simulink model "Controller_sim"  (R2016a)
settings: Solver=FixedStepAuto  StartTime=0.0  StopTime=Endtime  FixedStep=0.05  RelTol=1e-3
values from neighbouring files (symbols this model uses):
  alpha_A = (2^n - 1)/(V_A_max - V_A_min)    (= 204.6)    [Controller.m]    (also in ADConverter.m)
  alpha_i = 5/37.5    (= 0.133333333333)    [Controller.m]    (also in MotorDriver.m)
  alpha_T = 1.5/1000    (= 0.0015)    [Controller.m]    (also in Tachogenerator.m)
  d_i_d = (2^n-1)/60    (= 17.05)    [Controller.m]
  d_N_d = (2^n-1)/60    (= 17.05)    [Controller.m]
  m = 8    [Controller.m]    (also in PulseGenerator.m)
  u_max = 100    [Controller.m]    (also in SystemModel_noise1.m; SystemModel_noise2.m)
  u_min = 0    [Controller.m]    (also in SystemModel_noise1.m; SystemModel_noise2.m)
  V_A_min = 0    [Controller.m]    (also in ADConverter.m)
libraries: simulink x2

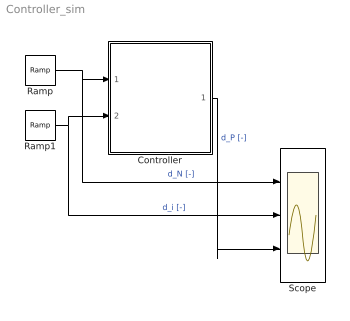
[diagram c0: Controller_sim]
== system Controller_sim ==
  Controller : Subsystem
  Ramp : simulink/Sources/Ramp  slope=d_N_d  start=0  X0=0
  Ramp1 : simulink/Sources/Ramp  slope=d_i_d  start=0  X0=0
  Scope : Scope  NumInputPorts=3
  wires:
  Ramp/1 -> Controller/1(d_N [-]), Scope/1  "d_N [-]"
  Controller/1(d_P [-]) -> Scope/3  "d_P [-]"
  Ramp1/1 -> Controller/2(d_i [-]), Scope/2  "d_i [-]"

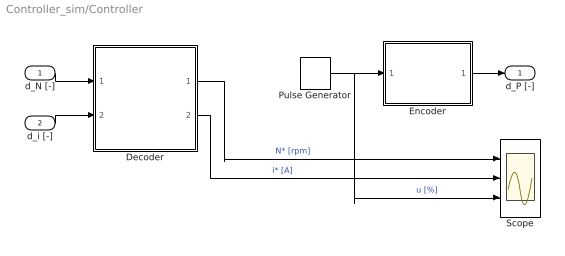
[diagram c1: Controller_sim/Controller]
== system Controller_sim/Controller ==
  d_N [-] : Inport
  d_i [-] : Inport  Port=2
  Decoder : Subsystem
  Encoder : Subsystem
  Pulse Generator : DiscretePulseGenerator  PulseType=Time based  Amplitude=100  Period=30  PulseWidth=50
  Scope : Scope  NumInputPorts=3
  d_P [-] : Outport
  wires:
  d_N [-]/1 -> Decoder/1(d_N [-])
  Encoder/1(d_P [-]) -> d_P [-]/1
  Decoder/1(N* [rpm]) -> Scope/1  "N* [rpm]"
  Decoder/2(i* [A]) -> Scope/2  "i* [A]"
  d_i [-]/1 -> Decoder/2(d_i [-])
  Pulse Generator/1 -> Scope/3, Encoder/1(u [%])  "u [%]"

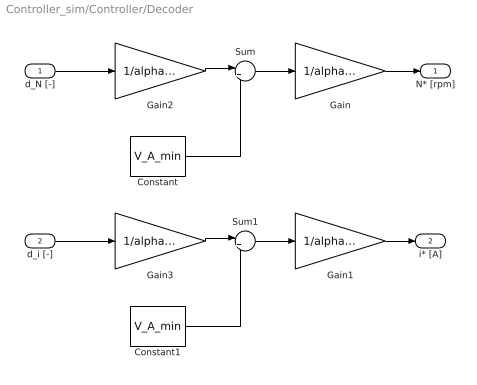
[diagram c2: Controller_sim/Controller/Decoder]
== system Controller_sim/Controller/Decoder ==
  d_N [-] : Inport
  d_i [-] : Inport  Port=2
  Constant : Constant  Value=V_A_min
  Constant1 : Constant  Value=V_A_min
  Gain : Gain  Gain=1/alpha_T
  Gain1 : Gain  Gain=1/alpha_i
  Gain2 : Gain  Gain=1/alpha_A
  Gain3 : Gain  Gain=1/alpha_A
  Sum : Sum  Inputs=|++
  Sum1 : Sum  Inputs=|++
  N* [rpm] : Outport
  i* [A] : Outport  Port=2
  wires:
  Gain/1 -> N* [rpm]/1
  d_N [-]/1 -> Gain2/1
  Sum/1 -> Gain/1
  Constant/1 -> Sum/2
  Gain2/1 -> Sum/1
  Gain1/1 -> i* [A]/1
  d_i [-]/1 -> Gain3/1
  Sum1/1 -> Gain1/1
  Constant1/1 -> Sum1/2
  Gain3/1 -> Sum1/1

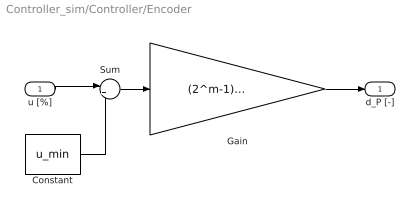
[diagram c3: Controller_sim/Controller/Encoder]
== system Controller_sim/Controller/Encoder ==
  u [%] : Inport
  Constant : Constant  Value=u_min
  Gain : Gain  Gain=(2^m-1)/(u_max-u_min)
  Sum : Sum  Inputs=|++
  d_P [-] : Outport
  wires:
  u [%]/1 -> Sum/1
  Gain/1 -> d_P [-]/1
  Sum/1 -> Gain/1
  Constant/1 -> Sum/2
